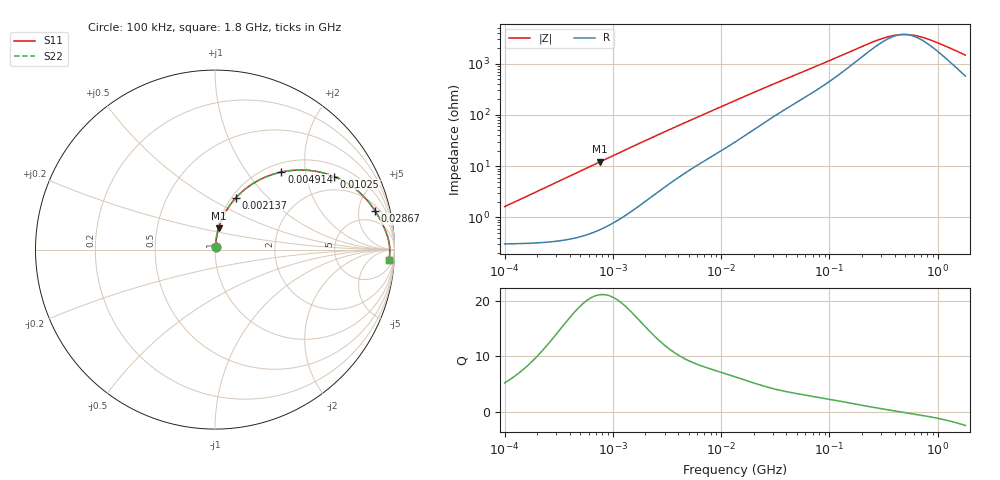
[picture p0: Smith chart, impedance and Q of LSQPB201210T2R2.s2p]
! LSQPB201210T2R2  S-PARAMETER MODEL  ( General Type )
! Model Generated by TAIYO YUDEN Corporation (http://www.ty-top.com)
! Version 2.0
! TAIYO YUDEN Control No. 100810NF18SB-HKC
! Copyright(c) 2007 TAIYO YUDEN CO.,LTD. All Rights Reserved.
! Product Description (link to TY-COMPAS)
! https://ds.yuden.co.jp/TYCOMPAS/or/detail?pn=LSQPB201210T2R2M&u=M
! Products Name : Inductors
! Characteristics :
!  Inductance : 2.2 uH , SRF(min) : 200 MHz , DC Resistance(max) : 0.39 Ohm
!  Rated Current : Saturation :600 mA , Temp Rise : 550 mA (40 degC)
!  Case Size : 2.0 x 1.25 / 0.079 x 0.049 [mm/inch] , Thickness : 1.0 / 0.04 [mm/inch]
!  (Conditions: Temperature = 25 degC , DC Bias Current/Voltage = 0A / 0V)
! External Node Assignments :
!  1  o---GGG---o  2
! GND o---------o GND
! Frequency Range : 0.1MHz  -  1800MHz  [ 402 STEP ]
# MHz S RI R 50
! Freq[MHz].  S11 Real  S11 Imag  S21 Real  S21 Imag  S12 Real  S12 Imag  S22 Real  S22 Imag
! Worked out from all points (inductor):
!   401 points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, 100 kHz to 1.8 GHz, reference 50 ohm
!   read as one part in series: L = 2.55 uH near 105 kHz
!   highest Q = 21 at 763.8 kHz (marker M1), where L = 2.54 uH
!   self-resonance near 483 MHz
!   S11 on the Smith chart (normalised r, x): 100 kHz: 1.01, +0.03; 2.137 MHz: 1.05, +0.67; 4.914 MHz: 1.16, +1.48; 10.25 MHz: 1.41, +2.92; 28.67 MHz: 2.70, +7.38; 1.8 GHz: 12, -27
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0.1  0.00329 0.0159  0.9967 -0.0159  0.9967 -0.0159  0.00329 0.0159
0.253659  0.00493 0.0403  0.9951 -0.0403  0.9951 -0.0403  0.00493 0.0403
0.516129  0.011 0.0813  0.989 -0.0813  0.989 -0.0813  0.011 0.0813
0.763781  0.0202 0.1189  0.9798 -0.1189  0.9798 -0.1189  0.0202 0.1189
1.341675  0.0534 0.1997  0.9466 -0.1997  0.9466 -0.1997  0.0534 0.1997
2.136843  0.1178 0.2901  0.8822 -0.2901  0.8822 -0.2901  0.1178 0.2901
2.66389  0.1666 0.3358  0.8334 -0.3358  0.8334 -0.3358  0.1666 0.3358
3.574164  0.2529 0.3911  0.7471 -0.3911  0.7471 -0.3911  0.2529 0.3911
4.914404  0.3702 0.4321  0.6298 -0.4321  0.6298 -0.4321  0.3702 0.4321
7.096489  0.5212 0.4415  0.4788 -0.4415  0.4788 -0.4415  0.5212 0.4415
10.24746  0.6642 0.407  0.3358 -0.407  0.3358 -0.407  0.6642 0.407
13.41641  0.7505 0.3612  0.2495 -0.3612  0.2495 -0.3612  0.7505 0.3612
19.37354  0.8357 0.2884  0.1643 -0.2884  0.1643 -0.2884  0.8357 0.2884
28.66948  0.8915 0.2165  0.1085 -0.2165  0.1085 -0.2165  0.8915 0.2165
69.24595  0.9497 0.1054  0.0503 -0.1054  0.0503 -0.1054  0.9497 0.1054
235.6695  0.9717 0.0266  0.0283 -0.0266  0.0283 -0.0266  0.9717 0.0266
357.3983  0.9732 0.0105  0.0268 -0.0105  0.0268 -0.0105  0.9732 0.0105
424.248  0.9735 0.00448  0.0265 -0.00448  0.0265 -0.00448  0.9735 0.00448
491.4156  0.9737 -0.000594  0.0263 0.000594  0.0263 0.000594  0.9737 -0.000594
659.3364  0.9737 -0.0109  0.0263 0.0109  0.0263 0.0109  0.9737 -0.0109
929.0554  0.9733 -0.0242  0.0267 0.0242  0.0267 0.0242  0.9733 -0.0242
1800  0.9703 -0.0595  0.0297 0.0595  0.0297 0.0595  0.9703 -0.0595
